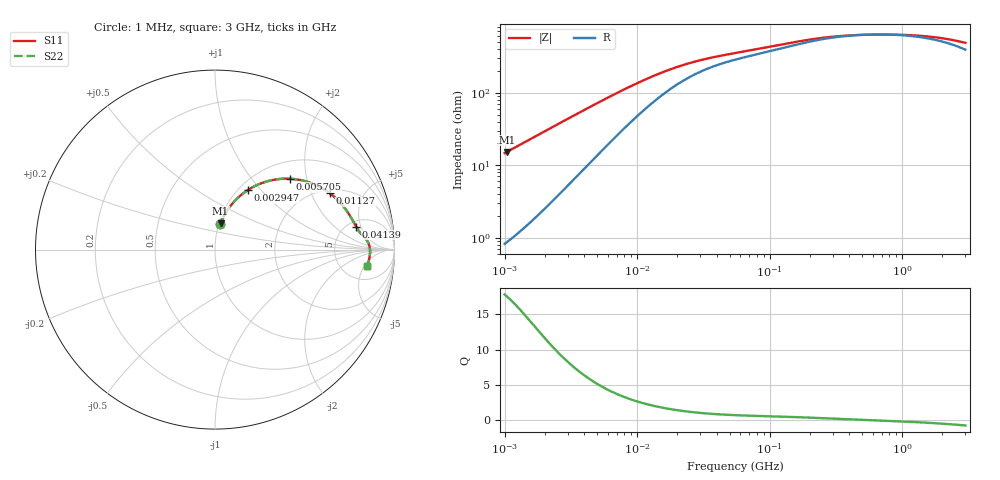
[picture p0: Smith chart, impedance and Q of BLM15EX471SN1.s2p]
! BLM15EX471SN1
# Hz S RI R 50
!Freq.(Hz) S11(Real) S11(Imag) S21(Real) S21(Imag) S12(Real) S12(Imag) S22(Real) S22(Imag)
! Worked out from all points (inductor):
!   401 points, 1 MHz to 3 GHz, reference 50 ohm
!   read as one part in series: L = 2.33 uH near 1.041 MHz
!   highest Q = 17.5 at 1.041 MHz (marker M1), where L = 2.33 uH
!   self-resonance near 617.2 MHz
!   S11 on the Smith chart (normalised r, x): 1 MHz: 1.02, +0.29; 2.947 MHz: 1.10, +0.85; 5.705 MHz: 1.35, +1.59; 11.27 MHz: 2.15, +2.75; 41.39 MHz: 5.89, +4.11; 3 GHz: 9, -6
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1000000  0.0287 0.1412  0.9713 -0.1412  0.9713 -0.1412  0.0287 0.1412
1040844  0.0308 0.1465  0.9692 -0.1465  0.9692 -0.1465  0.0308 0.1465
1405328  0.0525 0.1922  0.9475 -0.1922  0.9475 -0.1922  0.0525 0.1922
1822989  0.083 0.2389  0.917 -0.2389  0.917 -0.2389  0.083 0.2389
2317916  0.1249 0.2858  0.8751 -0.2858  0.8751 -0.2858  0.1249 0.2858
2947212  0.1828 0.3316  0.8172 -0.3316  0.8172 -0.3316  0.1828 0.3316
3823119  0.2646 0.3721  0.7354 -0.3721  0.7354 -0.3721  0.2646 0.3721
4670311  0.3382 0.3907  0.6618 -0.3907  0.6618 -0.3907  0.3382 0.3907
5705239  0.416 0.3949  0.584 -0.3949  0.584 -0.3949  0.416 0.3949
7703107  0.5278 0.3737  0.4722 -0.3737  0.4722 -0.3737  0.5278 0.3737
1.126754e7  0.6399 0.3142  0.3601 -0.3142  0.3601 -0.3142  0.6399 0.3142
1.461624e7  0.6931 0.2665  0.3069 -0.2665  0.3069 -0.2665  0.6931 0.2665
2.459509e7  0.7552 0.1829  0.2448 -0.1829  0.2448 -0.1829  0.7552 0.1829
4.138676e7  0.7859 0.1276  0.2141 -0.1276  0.2141 -0.1276  0.7859 0.1276
5.477226e7  0.798 0.108  0.202 -0.108  0.202 -0.108  0.798 0.108
2.094008e8  0.8505 0.0448  0.1495 -0.0448  0.1495 -0.0448  0.8505 0.0448
3.973271e8  0.8612 0.0172  0.1388 -0.0172  0.1388 -0.0172  0.8612 0.0172
8.005644e8  0.864 -0.0103  0.136 0.0103  0.136 0.0103  0.864 -0.0103
1.171007e9  0.8632 -0.0268  0.1368 0.0268  0.1368 0.0268  0.8632 -0.0268
1.645649e9  0.8608 -0.0447  0.1392 0.0447  0.1392 0.0447  0.8608 -0.0447
2.177892e9  0.8569 -0.0628  0.1431 0.0628  0.1431 0.0628  0.8569 -0.0628
3e9  0.8486 -0.0886  0.1514 0.0886  0.1514 0.0886  0.8486 -0.0886
